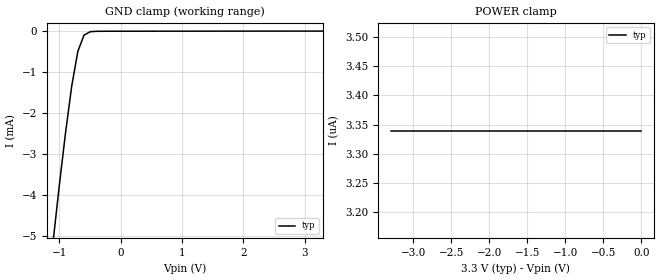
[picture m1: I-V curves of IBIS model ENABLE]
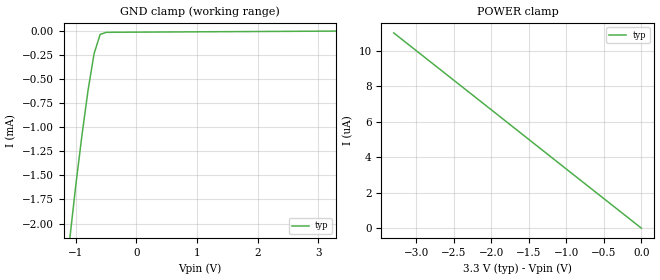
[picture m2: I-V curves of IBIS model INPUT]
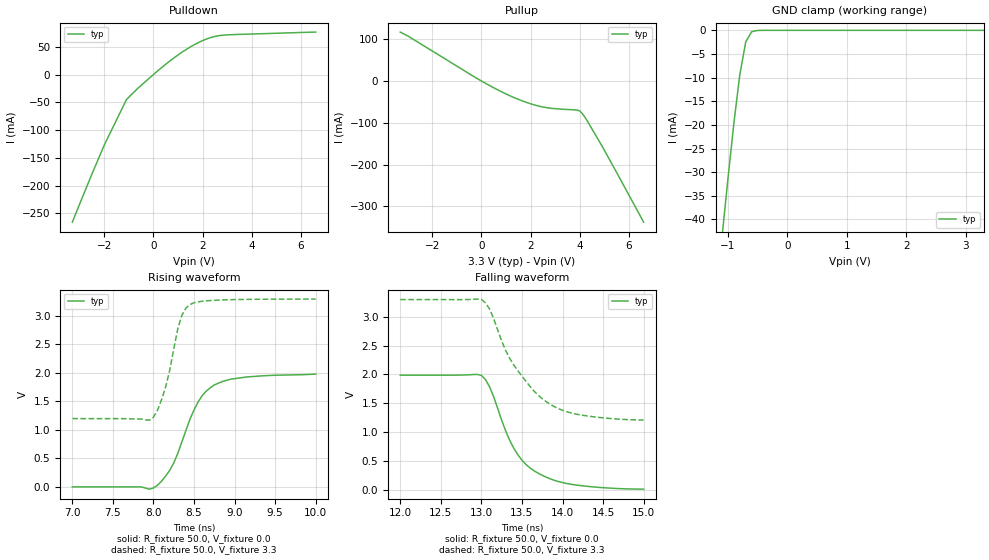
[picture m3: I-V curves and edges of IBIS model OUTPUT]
|   Texas Instruments Incorporated
|   Data Transmissions Products
|   IBIS Model for SN65LVDS048A
|   16PW TSSOP Package
[IBIS Ver]   3.2
[Comment char]   |_char
[File name]   lvds048apw.ibs
[File Rev]   2.0
[Date]   6Oct00
[Source]   File originated at Texas Instruments Incorporated.
   Data Transmission Products Group.
[Notes]
[Disclaimer]
(C) Copyright Texas Instruments Incorporated 2000
   All rights reserved
  Texas Instruments Incorporated hereby grants the user of this IBIS
model a non-exclusive, nontransferable license to use this IBIS model
under the following terms.  Before using this IBIS model, the user
should read this license.  If the user does not accept these terms,
the IBIS model should be returned to Texas Instruments within 30 days.
  The user is granted this license only to use the IBIS model and
is not granted rights to sell, load, rent, lease or license the IBIS
model in whole or in part, or in modified form to anyone other than
user.  User may modify the IBIS model to suit its specific applications
but rights to derivative works and such modifications shall belong to
Texas Instruments.
  This IBIS model is provided on an "AS IS" basis and Texas Instruments
makes absolutely no warranty with respect to the information contained
herein.  TEXAS INSTRUMENTS DISCLAIMS AND CUSTOMER WAIVES ALL WARRANTIES,
EXPRESS OR IMPLIED, INCLUDING WARRANTIES OF MERCHANTABILITY OR FITNESS
FOR A PARTICULAR PURPOSE. The entire risk as to quality and performance
is with the Customer. ACCORDINGLY, IN NO EVENT SHALL THE COMPANY BE LIABLE
FOR ANY DAMAGES, WHETHER IN CONTRACT OR TORT,INCLUDING ANY LOST PROFITS
OR OTHER INCIDENTAL, CONSEQUENTIAL, EXEMPLARY, OR PUNITIVE DAMAGES ARISING
OUT OF THE USE OR APPLICATION OF THE IBIS model provided in this package.
Further, Texas Instruments reserves the right to discontinue or make changes
without notice to any product herein to improve reliability, function, or
design. Texas Instruments does not convey any license under patent rights
or any other intellectual property rights, including those of third parties.
Contact Texas Instruments at ATTN:DATA TRANSMISSIONS
[Copyright]   Copyright 2000, Texas Instruments, All Rights Reserved
[Component]   SN65LVDS048APW
[Manufacturer]  Texas Instruments Incorporated
[Package]
|   typ   min   max
R_pkg   0.045   0.038   0.051
L_pkg   2.593nH   2.447nH   3.080nH
C_pkg   0.281pF   0.243pF   0.377pF
[Pin]   signal_name   model_name   R_pin   L_pin   C_pin
1   RIN1-   INPUT   0.040   3.080n   0.377p
2   RIN1+   INPUT   0.038   2.458n   0.281p
3   RIN2+   INPUT   0.051   2.512n   0.255p
4   RIN2-   INPUT   0.051   2.447n   0.243p
5   RIN3-   INPUT   0.051   2.447n   0.243p
6   RIN3+   INPUT   0.051   2.512n   0.255p
7   RIN4+   INPUT   0.038   2.458n   0.281p
8   RIN4-   INPUT   0.040   3.080n   0.377p
9   /EN   ENABLE   0.039   2.832n   0.316p
10   ROUT4   OUTPUT   0.038   2.460n   0.279p
11   ROUT3   OUTPUT   0.051   2.512n   0.255p
12   GND   GND   0.051   2.447n   0.243p
13   VCC   POWER   0.051   2.447n   0.243p
14   ROUT2   OUTPUT   0.051   2.512n   0.255p
15   ROUT1   OUTPUT   0.038   2.459n   0.279p
16   EN   ENABLE   0.039   2.832n   0.316p
[Diff_pin]   inv_pin   vdiff   tdelay_typ   tdelay_min   tdelay_max
| The 'RIN+' pin is Diff_pin and the 'RIN-' pin is the inv_pin
2   1   100mV   0 0 0   | Vth  +/-100mV
3   4   100mV   0 0 0
6   5   100mV   0 0 0
7   8   100mV   0 0 0
| Models and submodels in the file (3): ENABLE (Input), INPUT (Input), OUTPUT (3-state)
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|   Enable Model
[Model]   ENABLE
Model_type   Input
|Signals   /EN, EN
Vinh = 2.0
Vinl = 0.8
|   typ   min   max
C_comp   1.0pF   NA   NA
|   typ   min   max
[Temperature Range]   25.0   NA   NA
[Voltage range]   3.3V   3.0V   3.6V
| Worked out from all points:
|   GND clamp passes 1 mA (typ) near -0.76 V on its own axis
[GND_clamp]
|   Voltage   I(typ)   I(min)   I(max)
-3.3V     -43.1mA    NA         NA
-1.1V     -5.08mA    NA         NA
-1V       -3.73mA    NA         NA
-900mV    -2.47mA    NA         NA
-800mV    -1.34mA    NA         NA
-700mV    -493uA     NA         NA
-600mV    -98.5uA    NA         NA
-500mV    -13.3uA    NA         NA
3.3V      3.34uA     NA         NA
[Power_clamp]
| Note that the[POWER_clamp]voltage table is referenced to Vcc
| and is calculated using Vtable=Vcc - Vmeasured.
|   Voltage   I(typ)   I(min)   I(max)
-3.3V     3.34uA     NA         NA
-2.7V     3.34uA     NA         NA
-2V       3.34uA     NA         NA
-800mV    3.34uA     NA         NA
0V        3.34uA     NA         NA
|   Receiver Input Model
[Model]   INPUT
Model_type   Input
|Signals   RIN1-,RIN1+,RIN2+,RIN2-,RIN3-,RIN3+,RIN4+,RIN4-
Vinh = 2.0
Vinl = 0.8
|   typ   min   max
C_comp   1.0pF   NA   NA
|   typ   min   max
[Temperature Range]   25.0   NA   NA
[Voltage range]   3.3V   3.0V   3.6V
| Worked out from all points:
|   GND clamp passes 1 mA (typ) near -0.88 V on its own axis
[GND_clamp]
|   Voltage   I(typ)   I(min)   I(max)
-3.3V     -22.5mA    NA         NA
-1.1V     -2.15mA    NA         NA
-1V       -1.59mA    NA         NA
-900mV    -1.08mA    NA         NA
-800mV    -616uA     NA         NA
-700mV    -234uA     NA         NA
-600mV    -34.5uA    NA         NA
-500mV    -13.2uA    NA         NA
-400mV    -12.3uA    NA         NA
3.3V      8.31pA     NA         NA
[Power_clamp]
| Note that the[POWER_clamp]voltage table is referenced to Vcc
| and is calculated using Vtable=Vcc - Vmeasured.
|   Voltage   I(typ)   I(min)   I(max)
-3.3V     11uA       NA         NA
-3V       10uA       NA         NA
-2V       6.67uA     NA         NA
-1V       3.33uA     NA         NA
0V        8.31pA     NA         NA
|   Receiver Output Model
[Model]   OUTPUT
Model_type   3-state
| Signals   A1Y,A2Y,A3Y,A4Y,B1Y,B2Y,B3Y,B4Y,C1Y,C2Y,C3Y,C4Y,D1Y,D2Y,D3Y,D4Y
Vmeas = 1.5V   |Reference voltage for timing measurements
Cref = 8pF   |Timing specification test load capacitance value
Vref = 0   |Timing specification test load voltage; GND
| variable   typ   min   max
C_comp   1.0pF   NA   NA
|   typ   min   max
[Temperature Range]   25.0   NA   NA
[Voltage range]   3.3V   3.0V   3.6V
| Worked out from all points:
|   slope of the pulldown table from 0 to 0.495 V, typ, clamps not added: 26.9 ohm
|   slope of the pullup table from 0 to 0.495 V, typ, clamps not added: 30.7 ohm
|   GND clamp passes 1 mA (typ) near -0.63 V on its own axis
|   rising waveform, R_fixture 50.0, V_fixture 0.0: 20-80 % time 352ps typ, NA min, NA max; typ from 0 V to 1.98 V
|   falling waveform, R_fixture 50.0, V_fixture 0.0: 20-80 % time 420ps typ, NA min, NA max; typ from 1.99 V to 0.006 V
|   rising waveform, R_fixture 50.0, V_fixture 3.3: 20-80 % time 202ps typ, NA min, NA max; typ from 1.2 V to 3.3 V
|   falling waveform, R_fixture 50.0, V_fixture 3.3: 20-80 % time 538ps typ, NA min, NA max; typ from 3.3 V to 1.21 V
[Pulldown]
|   Voltage   I(typ)   I(min)   I(max)
-3.3V     -266mA     NA         NA
-2.5V     -179mA     NA         NA
-2V       -127mA     NA         NA
-1.1V     -45.3mA    NA         NA
-600mV    -23.5mA    NA         NA
600mV     22.1mA     NA         NA
1.2V      41.4mA     NA         NA
1.7V      54.7mA     NA         NA
2.1V      63mA       NA         NA
2.5V      68.7mA     NA         NA
3V        71.5mA     NA         NA
6.6V      76.5mA     NA         NA
[Pullup]
|   Voltage   I(typ)   I(min)   I(max)
| Note that the[Pullup]voltage table is referenced to Vcc
| and is calculated using Vtable=Vcc - Vmeasured.
-3.3V     117mA      NA         NA
-3V       108mA      NA         NA
0V        1.74nA     NA         NA
1.3V      -39mA      NA         NA
1.9V      -52.6mA    NA         NA
2.4V      -61mA      NA         NA
3.9V      -69.6mA    NA         NA
4V        -71.8mA    NA         NA
4.1V      -77.6mA    NA         NA
4.3V      -94.9mA    NA         NA
4.9V      -155mA     NA         NA
6.6V      -338mA     NA         NA
[GND_clamp]
|   Voltage   I(typ)   I(min)   I(max)
| Outputs in High Impedance (off)
-3.3V     -346mA     NA         NA
-1.1V     -43.9mA    NA         NA
-1V       -31.5mA    NA         NA
-900mV    -19.7mA    NA         NA
-800mV    -9.41mA    NA         NA
-700mV    -2.45mA    NA         NA
-600mV    -285uA     NA         NA
-400mV    -1.52uA    NA         NA
3.3V      489pA      NA         NA
[POWER_clamp]
|   Voltage   I(typ)   I(min)   I(max)
| Note that the [POWER_clamp] voltage table is referenced to Vcc
| and is calculated using Vtable = Vcc - Vmeasured.
| Outputs in Tri-state.
-3.3V     0A         NA         NA
0V        0A         NA         NA
[Ramp]
|   typ   min   max
dV/dt_r   1.20V/353ps   NA   NA
dV/dt_f   1.26V/540ps   NA   NA
R_load = 50
[Rising Waveform]
R_fixture = 50.0
V_fixture = 0.0
C_fixture = 0p
L_fixture = 0n
|   V(typ)   V(min)   V(max)
7ns       0V         NA         NA
8ns       -20mV      NA         NA
8.2ns     290mV      NA         NA
8.3ns     590mV      NA         NA
8.5ns     1.35V      NA         NA
8.6ns     1.6V       NA         NA
8.7ns     1.74V      NA         NA
8.85ns    1.85V      NA         NA
9.15ns    1.93V      NA         NA
10ns      1.98V      NA         NA
[Falling Waveform]
R_fixture = 50.0
V_fixture = 0.0
C_fixture = 0p
L_fixture = 0n
|   V(typ)   V(min)   V(max)
12ns      1.986V     NA         NA
13ns      1.982V     NA         NA
13.1ns    1.787V     NA         NA
13.3ns    1.016V     NA         NA
13.4ns    716mV      NA         NA
13.5ns    510mV      NA         NA
13.6ns    374mV      NA         NA
13.85ns   184mV      NA         NA
14.05ns   105mV      NA         NA
15ns      6mV        NA         NA
[Rising Waveform]
R_fixture = 50.0
V_fixture = 3.3
C_fixture = 0p
L_fixture = 0n
|   V(typ)   V(min)   V(max)
7ns       1.199V     NA         NA
7.95ns    1.171V     NA         NA
8ns       1.224V     NA         NA
8.05ns    1.349V     NA         NA
8.15ns    1.753V     NA         NA
8.3ns     2.778V     NA         NA
8.35ns    3.011V     NA         NA
8.45ns    3.201V     NA         NA
8.8ns     3.279V     NA         NA
10ns      3.297V     NA         NA
[Falling Waveform]
R_fixture = 50.0
V_fixture = 3.3
C_fixture = 0p
L_fixture = 0n
|   V(typ)   V(min)   V(max)
12ns      3.299V     NA         NA
13ns      3.303V     NA         NA
13.1ns    3.138V     NA         NA
13.25ns   2.58V      NA         NA
13.35ns   2.276V     NA         NA
13.6ns    1.789V     NA         NA
13.75ns   1.577V     NA         NA
13.95ns   1.404V     NA         NA
14.15ns   1.315V     NA         NA
15ns      1.206V     NA         NA
